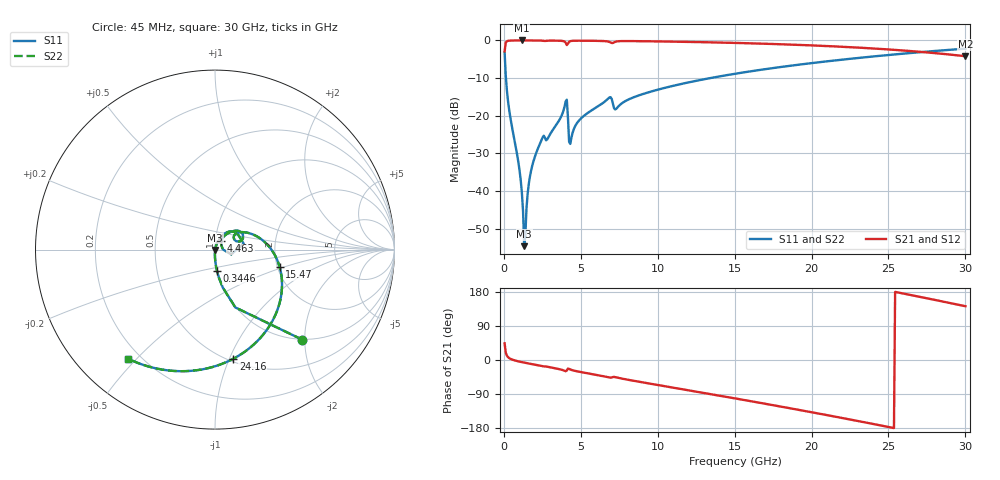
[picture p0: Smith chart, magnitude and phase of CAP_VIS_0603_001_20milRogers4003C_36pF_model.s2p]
! S-parameter model data by Modelithics Inc.  support@modelithics.com  813-866-6335  Tampa FL USA
! S-Parameter data specifications:
! Substrate: 20-mil Rogers 4003C, substrate thickness, H=0.508mm, Dielectric constant, Er=3.75
! PCB Mounting Pad Footprint: Pad width, PadW=0.90mm , Pad length, PadL=1.00mm , Pad gap, PadG (edge-to-edge)=1.00mm , Reference planes=3.0mm apart
! Created Wed Nov 18 13:28:19 2015
# hz S ma R 50
! 2 Port Network Data from SP1.SP block
! freq  magS11  angS11  magS21  angS21  magS12  angS12  magS22  angS22
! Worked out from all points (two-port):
!   401 points, 45 MHz to 30 GHz, reference 50 ohm
!   highest |S21| = -0.01 dB at 1.168 GHz (marker M1); lowest = -4.2 dB at 30 GHz (marker M2)
!   |S21| within 3 dB of the highest: start of sweep to 27.02 GHz
!   lowest |S11| = -54.6 dB at 1.318 GHz (marker M3), VSWR 1.00, Z = 50.1 - j0.156 ohm
!   |S11| at or under -10 dB: 132.7 MHz to 13.41 GHz (13.28 GHz wide, 196 % of centre)
!   |S22| runs from -54.6 to -2.2 dB; largest |S21 - S12| = 0
!   S11 on the Smith chart (normalised r, x): 45 MHz: 0.99, -1.95; 344.6 MHz: 0.99, -0.24; 4.463 GHz: 1.07, +0.10; 15.47 GHz: 2.06, -0.47; 24.16 GHz: 0.53, -1.03; 30 GHz: 0.15, -0.47
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4.5e7  0.6986 -45.9  0.7153 44.1  0.7153 44.1  0.6986 -45.9
3.4455e8  0.1186 -84.7  0.9923 5.0  0.9923 5.0  0.1186 -84.7
9.4365e8  0.02394 -91.2  0.9986 -3.6  0.9986 -3.6  0.02394 -91.2
1.168312e9  0.009509 -88.9  0.9987 -5.7  0.9987 -5.7  0.009509 -88.9
1.318088e9  0.001862 -57.0  0.9987 -6.9  0.9987 -6.9  0.001862 -57.0
1.467862e9  0.005914 69.5  0.9986 -8.1  0.9986 -8.1  0.005914 69.5
1.617638e9  0.0125 74.5  0.9984 -9.3  0.9984 -9.3  0.0125 74.5
1.8423e9  0.02181 75.0  0.9981 -11.0  0.9981 -11.0  0.02181 75.0
2.4414e9  0.04762 69.1  0.9944 -15.7  0.9944 -15.7  0.04762 69.1
3.93915e9  0.1317 50.4  0.9657 -28.3  0.9657 -28.3  0.1317 50.4
4.313588e9  0.0423 33.8  0.9771 -25.0  0.9771 -25.0  0.0423 33.8
4.463362e9  0.05936 53.2  0.9878 -27.1  0.9878 -27.1  0.05936 53.2
5.062462e9  0.09442 55.3  0.9911 -32.3  0.9911 -32.3  0.09442 55.3
6.784875e9  0.17 37.3  0.9643 -45.7  0.9643 -45.7  0.17 37.3
7.309088e9  0.1242 32.9  0.9675 -45.8  0.9675 -45.8  0.1242 32.9
1.007992e10  0.2242 22.6  0.9698 -66.5  0.9698 -66.5  0.2242 22.6
1.50225e10  0.3609 -11.9  0.9269 -101.3  0.9269 -101.3  0.3609 -11.9
1.547182e10  0.3734 -15.2  0.9218 -104.5  0.9218 -104.5  0.3734 -15.2
2.003996e10  0.5009 -48.7  0.8583 -138.1  0.8583 -138.1  0.5009 -48.7
2.415878e10  0.6168 -80.5  0.7784 -170.0  0.7784 -170.0  0.6168 -80.5
2.505742e10  0.6421 -87.7  0.7575 -177.2  0.7575 -177.2  0.6421 -87.7
3e10  0.7773 -128.6  0.6174 141.9  0.6174 141.9  0.7773 -128.6
